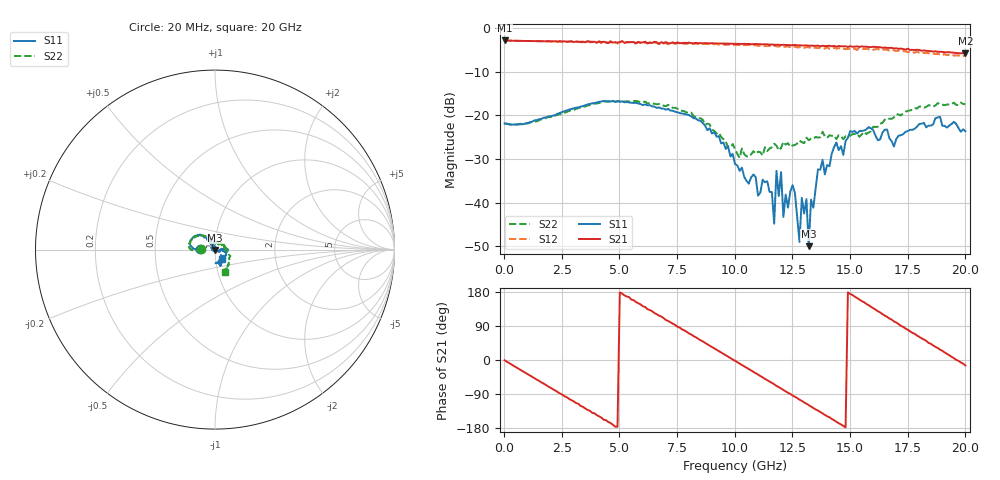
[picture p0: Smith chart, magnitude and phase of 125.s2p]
!Agilent Technologies,N5230A,US43500223,A.07.50.48
!Agilent N5230A: A.07.50.48
!Date: Thursday, October 08, 2015 16:59:21
!Correction: S11(Full 2 Port(1,2))
!S21(Full 2 Port(1,2))
!S12(Full 2 Port(1,2))
!S22(Full 2 Port(1,2))
!S2P File: Measurements: S11, S21, S12, S22:
# Hz S  RI  R 50
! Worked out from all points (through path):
!   201 points, 20 MHz to 20 GHz, reference 50 ohm
!   highest |S21| = -2.84 dB at 20 MHz (marker M1); lowest = -5.8 dB at 20 GHz (marker M2)
!   group delay of S21, straight-line fit = 102 ps
!   lowest |S11| = -49.9 dB at 13.21 GHz (marker M3), VSWR 1.01, Z = 50.2 - j0.277 ohm
!   |S11| at or under -10 dB: start of sweep to end of sweep
!   |S22| runs from -29.7 to -16.5 dB; largest |S21 - S12| = 0.065
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2e7  -0.081 0.00131  0.7211 -0.00957  0.7195 -0.0113  -0.0806 0.000872
1.9181e9  -0.0972 -0.00455  0.2413 -0.6668  0.2295 -0.6673  -0.0955 -0.009
3.4166e9  -0.127 0.0132  -0.3857 -0.5822  -0.3845 -0.564  -0.1257 -0.00363
5.1149e9  -0.1332 0.0562  -0.7069 0.0582  -0.6953 0.0741  -0.1453 0.0332
6.7133e9  -0.0948 0.0791  -0.3011 0.5865  -0.2809 0.5935  -0.1163 0.0683
8.3117e9  -0.0615 0.0687  0.3373 0.5864  0.3513 0.5646  -0.0561 0.0761
1.001e10  -0.0112 0.0254  0.6626 -0.0233  0.6429 -0.0524  0.000679 0.0413
1.14086e10  -0.0124 0.0125  0.3904 -0.5217  0.3525 -0.522  0.0222 0.0321
1.17083e10  -0.00384 0.00429  0.2809 -0.5777  0.2474 -0.5744  0.0311 0.0358
1.18082e10  -0.0216 0.00849  0.2371 -0.5984  0.1983 -0.5857  0.0336 0.0298
1.2008e10  -0.0186 0.0124  0.1629 -0.6185  0.1304 -0.612  0.0289 0.031
1.21079e10  -0.0035 0.00591  0.1271 -0.6315  0.0848 -0.6054  0.0344 0.036
1.25075e10  -0.0153 -0.00441  -0.0429 -0.635  -0.0603 -0.608  0.0366 0.0265
1.28072e10  -0.000104 -0.00355  -0.1613 -0.6135  -0.1705 -0.5792  0.0402 0.0324
1.29071e10  0.00816 -0.00791  -0.194 -0.603  -0.2241 -0.5642  0.0386 0.0307
1.31069e10  0.00515 -0.00971  -0.2712 -0.5727  -0.2764 -0.5373  0.0477 0.0286
1.32068e10  0.00158 -0.00276  -0.3043 -0.5482  -0.3288 -0.5058  0.047 0.0223
1.33067e10  -0.00371 -0.0102  -0.3403 -0.5299  -0.3398 -0.4822  0.0462 0.0282
1.34066e10  0.00702 -0.00523  -0.3717 -0.5051  -0.3736 -0.4673  0.0457 0.0284
1.44056e10  0.0488 -0.00275  -0.5844 -0.18  -0.5662 -0.1402  0.0526 0.0104
1.67033e10  0.0422 -0.0351  -0.1974 0.5591  -0.1705 0.5281  0.0801 -0.0444
2e10  0.0392 -0.0531  0.4956 -0.1263  0.4572 -0.1487  0.0556 -0.1222
